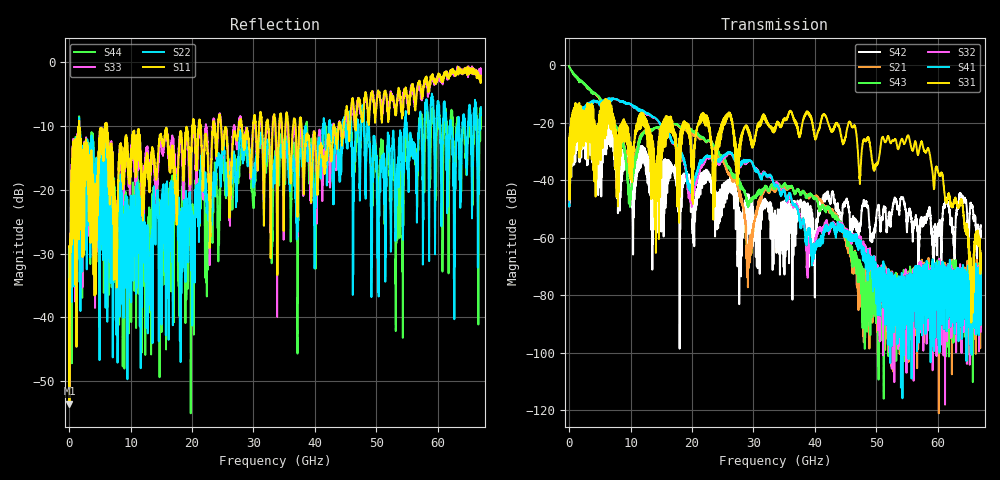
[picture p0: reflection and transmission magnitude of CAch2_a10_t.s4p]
!Agilent Technologies,N5247A,US51170199,A.09.90.13
!Agilent N5247A: A.09.90.13
!Date: Tuesday, October 23, 2018 14:34:30
!Correction: S11(Full 4 Port(1,2,3,4))
!S12(Full 4 Port(1,2,3,4))
!S13(Full 4 Port(1,2,3,4))
!S14(Full 4 Port(1,2,3,4))
!S21(Full 4 Port(1,2,3,4))
!S22(Full 4 Port(1,2,3,4))
!S23(Full 4 Port(1,2,3,4))
!S24(Full 4 Port(1,2,3,4))
!S31(Full 4 Port(1,2,3,4))
!S32(Full 4 Port(1,2,3,4))
!S33(Full 4 Port(1,2,3,4))
!S34(Full 4 Port(1,2,3,4))
!S41(Full 4 Port(1,2,3,4))
!S42(Full 4 Port(1,2,3,4))
!S43(Full 4 Port(1,2,3,4))
!S44(Full 4 Port(1,2,3,4))
!S4P File: Measurements: <S11,S12,S13,S14>,
!<S21,S22,S23,S24>,
!<S31,S32,S33,S34>,
!<S41,S42,S43,S44>:
# Hz S  dB  R 50
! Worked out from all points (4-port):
!   6701 points, 10 MHz to 67 GHz, reference 50 ohm
!   strongest paths, dB at 10 MHz, 16.76 GHz, 33.51 GHz, 50.25 GHz, 67 GHz:
!     S31: -33.3, -23.0, -21.6, -33.9, -67.4
!     S41: -48.7, -26.3, -41.8, -75.9, -74.0
!     S32: -48.5, -26.6, -41.4, -82.1, -92.7
!     S43: -0.3, -20.6, -42.7, -82.2, -78.7
!     S21: -0.4, -20.6, -43.6, -84.0, -74.6
!     S42: -33.5, -36.5, -50.8, -49.3, -55.6
!   lowest |S11| = -53.5 dB at 59.99 MHz (marker M1), VSWR 1.00, Z = 50.2 - j0.0111 ohm
!   |S11| at or under -10 dB: 1.645 GHz to 5.887 GHz (4.242 GHz wide, 113 % of centre); 6.191 GHz to 20.06 GHz (13.86 GHz wide, 106 % of centre); 37.84 GHz to 43.09 GHz (5.248 GHz wide, 13 % of centre)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
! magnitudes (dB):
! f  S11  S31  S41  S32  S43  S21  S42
! 10 MHz  -28.9  -33.3  -48.7  -48.5  -0.3  -0.4  -33.5
! 59.99 MHz  -53.5  -27.9  -47.7  -47.8  -0.7  -0.7  -28.5
! 7.549 GHz  -27.8  -26.3  -11.7  -11.8  -20.9  -21.0  -33.4
! 9.929 GHz  -17.3  -33.3  -13.4  -13.6  -49.3  -38.6  -36.1
! 19.58 GHz  -15.2  -22.5  -43.3  -46.4  -22.0  -22.8  -39.6
! 55.13 GHz  -6.9  -24.4  -85.8  -73.8  -80.9  -76.1  -53.1
! 67 GHz  -2.1  -67.4  -74.0  -92.7  -78.7  -74.6  -55.6
